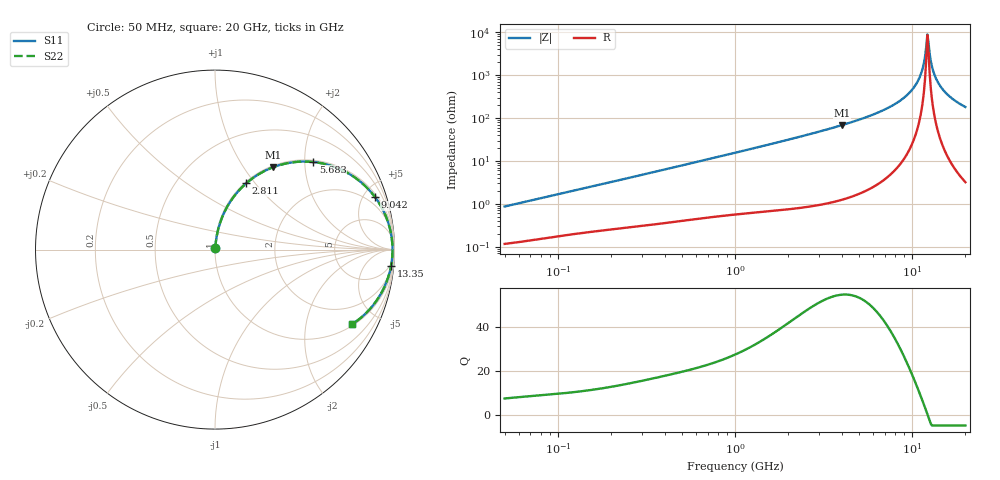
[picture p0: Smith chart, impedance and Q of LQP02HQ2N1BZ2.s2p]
!Murata Part Number: LQP02HQ2N1BZ2
!These Parameters are Measured in Series Mode Connection
!  o--[Z]--o
!Port1  Port2
!  o-------o
!Freq. Start=50[MHz] Stop=20[GHz], 401[Steps]
# Hz S RI R 50
!Freq.(Hz) S11(Real) S11(Imag) S21(Real) S21(Imag) S12(Real) S12(Imag) S22(Real) S22(Imag)
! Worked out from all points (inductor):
!   401 points, 50 MHz to 20 GHz, reference 50 ohm
!   read as one part in series: L = 2.71 nH near 51.52 MHz
!   highest Q = 55.1 at 4.027 GHz (marker M1), where L = 2.71 nH
!   self-resonance near 12.2 GHz
!   S11 on the Smith chart (normalised r, x): 50 MHz: 1.00, +0.02; 2.811 GHz: 1.02, +0.90; 5.683 GHz: 1.04, +2.20; 9.042 GHz: 1.23, +6.05; 13.35 GHz: 3, -21; 20 GHz: 1.06, -3.62
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5e7  0.00123 0.00856  0.9988 -0.00856  0.9988 -0.00856  0.00123 0.00856
1.364002e8  0.00257 0.0222  0.9974 -0.0222  0.9974 -0.0222  0.00257 0.0222
3.721004e8  0.0068 0.0581  0.9932 -0.0581  0.9932 -0.0581  0.0068 0.0581
1e9  0.0287 0.1497  0.9713 -0.1497  0.9713 -0.1497  0.0287 0.1497
2.728004e9  0.1653 0.3615  0.8347 -0.3615  0.8347 -0.3615  0.1653 0.3615
2.810964e9  0.1743 0.3696  0.8257 -0.3696  0.8257 -0.3696  0.1743 0.3696
4.026975e9  0.3234 0.4588  0.6766 -0.4588  0.6766 -0.4588  0.3234 0.4588
5.683258e9  0.5471 0.488  0.4529 -0.488  0.4529 -0.488  0.5471 0.488
7.442007e9  0.7576 0.416  0.2424 -0.416  0.2424 -0.416  0.7576 0.416
9.041845e9  0.8928 0.291  0.1072 -0.291  0.1072 -0.291  0.8928 0.291
1.019291e10  0.9522 0.1855  0.0478 -0.1855  0.0478 -0.1855  0.9522 0.1855
1.098561e10  0.976 0.1116  0.024 -0.1116  0.024 -0.1116  0.976 0.1116
1.149051e10  0.9846 0.0653  0.0154 -0.0653  0.0154 -0.0653  0.9846 0.0653
1.201863e10  0.9888 0.0182  0.0112 -0.0182  0.0112 -0.0182  0.9888 0.0182
1.220001e10  0.9892 0.00241  0.0108 -0.00241  0.0108 -0.00241  0.9892 0.00241
1.238412e10  0.9891 -0.0134  0.0109 0.0134  0.0109 0.0134  0.9891 -0.0134
1.257102e10  0.9884 -0.0291  0.0116 0.0291  0.0116 0.0291  0.9884 -0.0291
1.295331e10  0.9857 -0.0606  0.0143 0.0606  0.0143 0.0606  0.9857 -0.0606
1.334722e10  0.9809 -0.0917  0.0191 0.0917  0.0191 0.0917  0.9809 -0.0917
1.417136e10  0.9656 -0.1524  0.0344 0.1524  0.0344 0.1524  0.9656 -0.1524
1.550395e10  0.9293 -0.2374  0.0707 0.2374  0.0707 0.2374  0.9293 -0.2374
2e10  0.7628 -0.4167  0.2372 0.4167  0.2372 0.4167  0.7628 -0.4167
